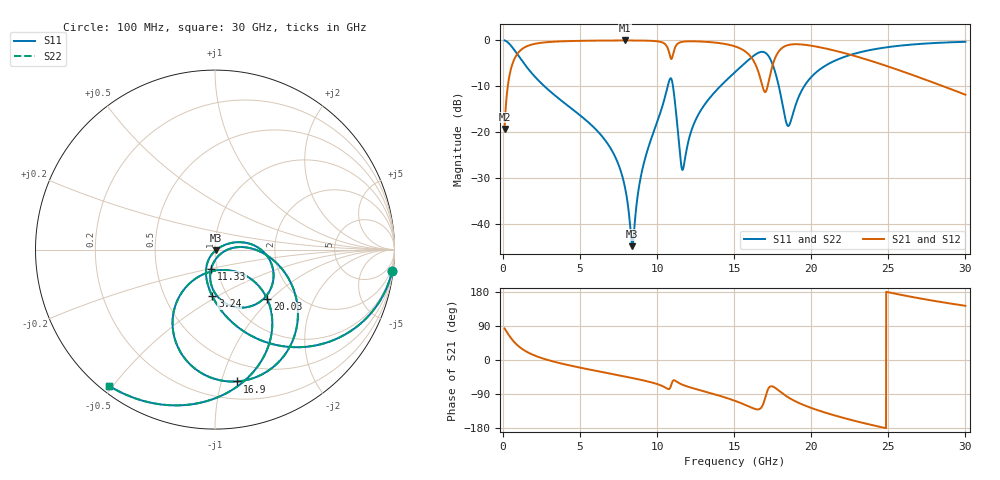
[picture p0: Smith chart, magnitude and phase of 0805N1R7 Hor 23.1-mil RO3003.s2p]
# GHz S MA R 50
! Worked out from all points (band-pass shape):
!   3201 points, 100 MHz to 30 GHz, reference 50 ohm
!   highest |S21| = -0.05 dB at 7.902 GHz (marker M1); lowest = -19.3 dB at 100 MHz (marker M2)
!   |S21| within 3 dB of the highest: 909.9 MHz to 10.8 GHz (9.895 GHz wide, 169 % of centre); 11.03 GHz to 15.93 GHz (4.899 GHz wide, 36.3 % of centre)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
!   lowest |S11| = -44.9 dB at 8.388 GHz (marker M3), VSWR 1.01, Z = 50.4 - j0.444 ohm
!   |S11| at or under -10 dB: 2.675 GHz to 10.68 GHz (8.009 GHz wide, 120 % of centre); 11.02 GHz to 14.1 GHz (3.079 GHz wide, 24.5 % of centre); 17.89 GHz to 19.54 GHz (1.653 GHz wide, 8.83 % of centre)
!   |S22| runs from -44.9 to -0.1 dB; largest |S21 - S12| = 0
!   S11 on the Smith chart (normalised r, x): 100 MHz: 1, -17; 3.24 GHz: 0.85, -0.47; 11.33 GHz: 0.94, -0.20; 16.9 GHz: 0.34, -1.12; 20.03 GHz: 1.45, -0.96; 30 GHz: 0.02, -0.49
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0.1  0.9941 -6.8  0.1082 83.2  0.1082 83.2  0.9941 -6.8
0.4270312  0.9066 -27.4  0.4215 62.5  0.4215 62.5  0.9066 -27.4
0.8755312  0.7228 -48.8  0.6902 41.2  0.6902 41.2  0.7228 -48.8
3.2395  0.2608 -93.2  0.963 -3.8  0.963 -3.8  0.2608 -93.2
5.089563  0.1478 -109.7  0.9857 -20.9  0.9857 -20.9  0.1478 -109.7
7.902031  0.02539 -122.2  0.9944 -43.6  0.9944 -43.6  0.02539 -122.2
8.387906  0.005715 -50.4  0.994 -47.6  0.994 -47.6  0.005715 -50.4
9.023281  0.03818 25.9  0.9917 -53.1  0.9917 -53.1  0.03818 25.9
10.06978  0.1392 17.4  0.9702 -64.4  0.9702 -64.4  0.1392 17.4
10.87334  0.3856 -43.9  0.6401 -70.6  0.6401 -70.6  0.3856 -43.9
11.33119  0.108 -101.3  0.9173 -58.8  0.9173 -58.8  0.108 -101.3
11.67691  0.03945 -37.3  0.9647 -65.8  0.9647 -65.8  0.03945 -37.3
12.70472  0.1586 5.0  0.9702 -78.9  0.9702 -78.9  0.1586 5.0
15.05  0.4494 -22.4  0.8569 -107.7  0.8569 -107.7  0.4494 -22.4
16.18059  0.6616 -48.7  0.6249 -126.7  0.6249 -126.7  0.6616 -48.7
16.90006  0.7448 -80.5  0.2898 -113.9  0.2898 -113.9  0.7448 -80.5
17.57281  0.4986 -118.1  0.5897 -71.3  0.5897 -71.3  0.4986 -118.1
18.4885  0.1164 -85.3  0.8856 -98.2  0.8856 -98.2  0.1164 -85.3
20.03022  0.4025 -43.5  0.8699 -127.0  0.8699 -127.0  0.4025 -43.5
20.03956  0.404 -43.6  0.8694 -127.1  0.8694 -127.1  0.404 -43.6
25.01978  0.8436 -92.8  0.5154 178.6  0.5154 178.6  0.8436 -92.8
30  0.9616 -127.9  0.2552 143.0  0.2552 143.0  0.9616 -127.9
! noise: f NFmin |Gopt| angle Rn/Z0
0.1  0.001061  0.945  1.495  0.004317
3.417  0.006975  0.729  20.63  0.004963
6.743  0.01238  0.7091  38.93  0.007469
10.06  0.0328  0.8305  56.29  0.03178
13.39  0.03499  0.7999  72.81  0.02363
16.7  0.2922  0.9685  88.7  1.074
20.03  0.071  0.8576  103.1  0.04162
23.35  0.06434  0.8262  115.9  0.02242
26.67  0.07573  0.8374  128.2  0.01944
30  0.09794  0.8642  140.2  0.01864
